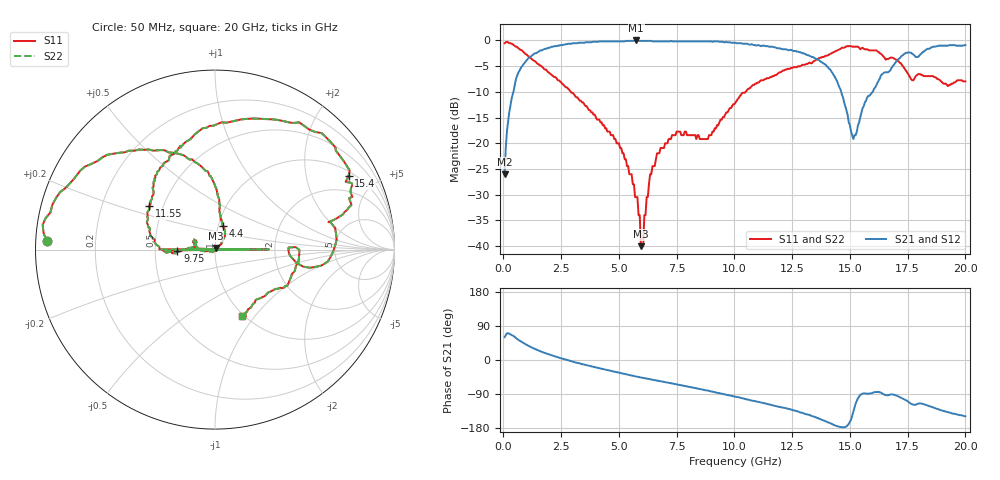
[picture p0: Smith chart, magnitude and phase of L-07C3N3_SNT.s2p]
#	mhz	s	ma	r	50
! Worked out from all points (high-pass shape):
!   400 points, 50 MHz to 20 GHz, reference 50 ohm
!   highest |S21| = 0.00 dB at 5.75 GHz (marker M1); lowest = -26.0 dB at 50 MHz (marker M2)
!   |S21| within 3 dB of the highest: 1.22 GHz to 13.26 GHz (12.04 GHz wide, 166 % of centre); 17.99 GHz to end of sweep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
!   lowest |S11| = -40.0 dB at 5.95 GHz (marker M3), VSWR 1.02, Z = 50.5 + j0.859 ohm
!   |S11| at or under -10 dB: 2.919 GHz to 10.48 GHz (7.563 GHz wide, 113 % of centre)
!   |S22| runs from -40.0 to -0.3 dB; largest |S21 - S12| = 0
!   S11 on the Smith chart (normalised r, x): 50 MHz: 0.03, +0.03; 4.4 GHz: 1.05, +0.29; 9.75 GHz: 0.65, -0.01; 11.55 GHz: 0.42, +0.25; 15.4 GHz: 1.18, +3.51; 20 GHz: 0.97, -0.86
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50  0.94 177.0  0.05 60.2  0.05 60.2  0.94 177.0
250  0.94 167.3  0.2 69.8  0.2 69.8  0.94 167.3
750  0.81 140.5  0.54 49.6  0.54 49.6  0.81 140.5
3400  0.25 84.1  0.95 -10.7  0.95 -10.7  0.25 84.1
4400  0.14 72.1  0.98 -25.0  0.98 -25.0  0.14 72.1
5750  0.03 43.9  1 -43.6  1 -43.6  0.03 43.9
5950  0.01 58.2  0.99 -46.0  0.99 -46.0  0.01 58.2
6700  0.08 -176.9  0.98 -55.0  0.98 -55.0  0.08 -176.9
9350  0.16 178.9  0.97 -87.5  0.97 -87.5  0.16 178.9
9400  0.17 -0.1  0.97 -88.1  0.97 -88.1  0.17 -0.1
9450  0.17 -179.1  0.97 -88.8  0.97 -88.8  0.17 -179.1
9750  0.21 -177.3  0.96 -93.1  0.96 -93.1  0.21 -177.3
10050  0.25 -177.5  0.95 -97.1  0.95 -97.1  0.25 -177.5
10250  0.29 -179.1  0.94 -99.6  0.94 -99.6  0.29 -179.1
10300  0.3 0.3  0.94 -100.4  0.94 -100.4  0.3 0.3
10350  0.31 179.7  0.93 -101.2  0.93 -101.2  0.31 179.7
11550  0.44 146.4  0.87 -117.9  0.87 -117.9  0.44 146.4
13350  0.6 108.7  0.69 -147.8  0.69 -147.8  0.6 108.7
14650  0.85 56.5  0.3 -177.2  0.3 -177.2  0.85 56.5
15400  0.85 28.9  0.16 -96.4  0.16 -96.4  0.85 28.9
16700  0.67 11.8  0.5 -92.0  0.5 -92.0  0.67 11.8
20000  0.4 -68.2  0.9 -148.5  0.9 -148.5  0.4 -68.2
